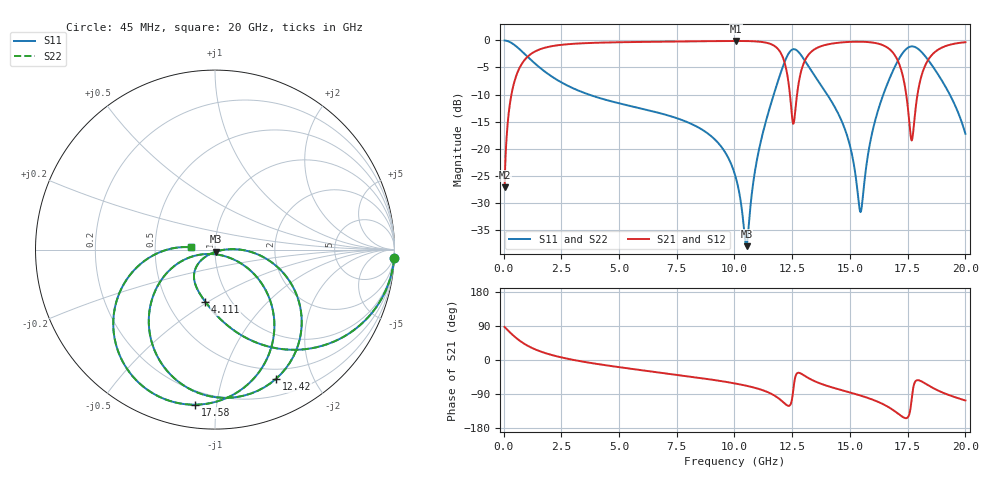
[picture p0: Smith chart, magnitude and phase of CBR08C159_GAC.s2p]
! S-parameter model data by Modelithics Inc.  support@modelithics.com 813-866-6335  Tampa FL USA
! S-Parameter data specifications:
! Substrate: 20-mil Rogers 4350B, substrate thickness, H=0.508mm, Dielectric constant, Er=3.75
! PCB Mounting Pad Footprint: Pad width, PadW=1.45mm , Pad length, PadL=1mm , Pad gap, PadG (edge-to-edge)=0.6mm , Reference planes=2.6mm apart
#  GHz  S  MA  R 50
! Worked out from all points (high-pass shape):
!   801 points, 45 MHz to 20 GHz, reference 50 ohm
!   highest |S21| = -0.10 dB at 10.05 GHz (marker M1); lowest = -27.1 dB at 45 MHz (marker M2)
!   |S21| within 3 dB of the highest: 1.019 GHz to 12.09 GHz (11.07 GHz wide, 169 % of centre); 13.13 GHz to 17 GHz (3.867 GHz wide, 25.7 % of centre)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
!   lowest |S11| = -38.0 dB at 10.52 GHz (marker M3), VSWR 1.03, Z = 50.5 - j1.15 ohm
!   |S11| at or under -10 dB: 3.69 GHz to 11.7 GHz (8.011 GHz wide, 104 % of centre); 14.01 GHz to 16.45 GHz (2.43 GHz wide, 16 % of centre); 19.32 GHz to end of sweep
!   |S22| runs from -38.0 to 0.0 dB; largest |S21 - S12| = 0
!   S11 on the Smith chart (normalised r, x): 45 MHz: 1, -40; 4.111 GHz: 0.76, -0.49; 12.42 GHz: 0.38, -1.51; 17.58 GHz: 0.12, -0.87; 20 GHz: 0.76, +0.02
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0.045  0.999 -2.8  0.04404 87.2  0.04404 87.2  0.999 -2.8
0.319381  0.9544 -19.6  0.2981 70.4  0.2981 70.4  0.9544 -19.6
0.793312  0.7924 -43.1  0.6092 46.9  0.6092 46.9  0.7924 -43.1
3.387462  0.3341 -93.5  0.9401 -3.8  0.9401 -3.8  0.3341 -93.5
4.110831  0.2956 -100.6  0.9526 -11.0  0.9526 -11.0  0.2956 -100.6
6.704981  0.2145 -121.8  0.9725 -32.7  0.9725 -32.7  0.2145 -121.8
10.0225  0.05725 -142.6  0.9882 -61.9  0.9882 -61.9  0.05725 -142.6
10.04744  0.05491 -142.4  0.9882 -62.2  0.9882 -62.2  0.05491 -142.4
10.52138  0.01255 -65.6  0.9864 -68.0  0.9864 -68.0  0.01255 -65.6
10.99531  0.08349 1.6  0.9767 -75.3  0.9767 -75.3  0.08349 1.6
11.74362  0.3386 -13.8  0.8854 -94.3  0.8854 -94.3  0.3386 -13.8
12.4171  0.7963 -64.7  0.2932 -118.3  0.2932 -118.3  0.7963 -64.7
12.59171  0.8297 -84.1  0.185 -57.6  0.185 -57.6  0.8297 -84.1
12.89103  0.7276 -111.4  0.5236 -36.1  0.5236 -36.1  0.7276 -111.4
13.36496  0.5106 -135.9  0.7986 -52.9  0.7986 -52.9  0.5106 -135.9
14.78676  0.1503 -162.9  0.9636 -82.0  0.9636 -82.0  0.1503 -162.9
15.46024  0.0259 -94.8  0.9727 -93.9  0.9727 -93.9  0.0259 -94.8
16.68248  0.4275 -43.4  0.8408 -124.8  0.8408 -124.8  0.4275 -43.4
17.23124  0.7366 -71.6  0.5239 -148.1  0.5239 -148.1  0.7366 -71.6
17.58046  0.8711 -97.2  0.1674 -141.1  0.1674 -141.1  0.8711 -97.2
18.27888  0.7065 -143.3  0.5993 -62.8  0.5993 -62.8  0.7065 -143.3
20  0.137 174.5  0.9623 -106.8  0.9623 -106.8  0.137 174.5
